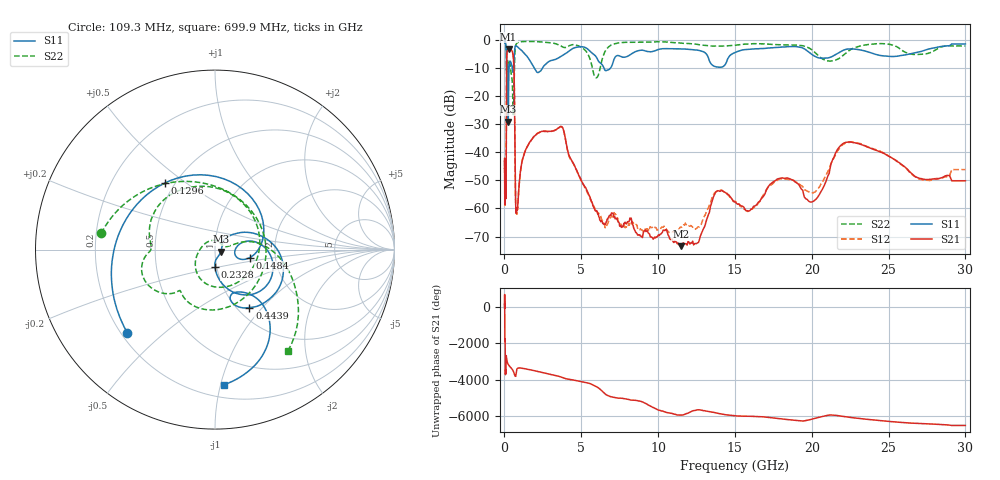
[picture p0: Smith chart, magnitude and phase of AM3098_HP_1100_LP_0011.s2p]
! Date/Time: Thu, Feb 28, 2019 8:44 AM
! Network Analyzer: Agilent Technologies E8364B Rev: A.07.50.67
! Sweep from 0.010 to 30.000 GHz, 1601 Points, Sweep Type: LOG
! Power Supply: 5.023 V, 0.002 A
# Hz S DB R 50
!freq MagS11 AngS11 MagS21 AngS21 MagS12 AngS12 MagS22 AngS22
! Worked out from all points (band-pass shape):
!   1601 points, 10 MHz to 30 GHz, reference 50 ohm
!   highest |S21| = -3.36 dB at 266.5 MHz (marker M1); lowest = -73.4 dB at 11.48 GHz (marker M2)
!   |S21| within 3 dB of the highest: 148.6 MHz to 580.7 MHz (432.2 MHz wide, 119 % of centre)
!   lowest |S11| = -29.2 dB at 246 MHz (marker M3), VSWR 1.07, Z = 53.4 - j1.21 ohm
!   |S11| at or under -10 dB: 204.7 MHz to 299.9 MHz (95.23 MHz wide, 37.7 % of centre); 1.921 GHz to 2.492 GHz (570.8 MHz wide, 25.9 % of centre); 6.469 GHz to 6.924 GHz (454.3 MHz wide, 6.78 % of centre)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
!   |S22| runs from -26.7 to -0.5 dB; largest |S21 - S12| = 0.012
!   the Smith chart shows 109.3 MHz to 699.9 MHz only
!   S11 on the Smith chart (normalised r, x): 109.3 MHz: 0.22, -0.38; 129.6 MHz: 0.44, +0.42; 148.4 MHz: 1.47, -0.14; 232.8 MHz: 0.98, -0.19; 443.9 MHz: 1.13, -0.85; 699.9 MHz: 0.29, -1.02
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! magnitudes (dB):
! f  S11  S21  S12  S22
! 10 MHz  -0.4  -45.9  -43.0  -0.5
! 38.04 MHz  -0.4  -55.7  -57.2  -0.7
! 109.3 MHz  -3.4  -51.3  -51.6  -3.9
! 129.6 MHz  -6.7  -21.4  -21.4  -10.7
! 144.7 MHz  -11.8  -7.6  -7.5  -9.5
! 148.4 MHz  -14.1  -6.4  -6.4  -10.0
! 232.8 MHz  -20.3  -3.5  -3.4  -8.8
! 246 MHz  -29.2  -3.4  -3.3  -8.9
! 266.5 MHz  -16.6  -3.4  -3.3  -8.9
! 443.9 MHz  -8.5  -3.8  -3.7  -12.4
! 550.5 MHz  -11.6  -5.1  -5.1  -24.5
! 630.1 MHz  -6.2  -12.9  -12.8  -13.6
! 699.9 MHz  -2.5  -48.3  -48.2  -3.1
! 801.2 MHz  -2.4  -60.4  -61.7  -1.4
! 2.084 GHz  -11.4  -33.7  -33.6  -0.7
! 3.723 GHz  -5.9  -30.9  -31.0  -2.4
! 7.926 GHz  -6.1  -65.5  -66.7  -1.0
! 11.48 GHz  -3.3  -73.4  -66.6  -1.3
! 14.02 GHz  -9.9  -53.9  -53.6  -2.3
! 20.2 GHz  -6.0  -57.1  -54.2  -4.6
! 22.56 GHz  -3.3  -36.4  -36.4  -3.5
! 30 GHz  -1.6  -50.2  -46.2  -2.3
